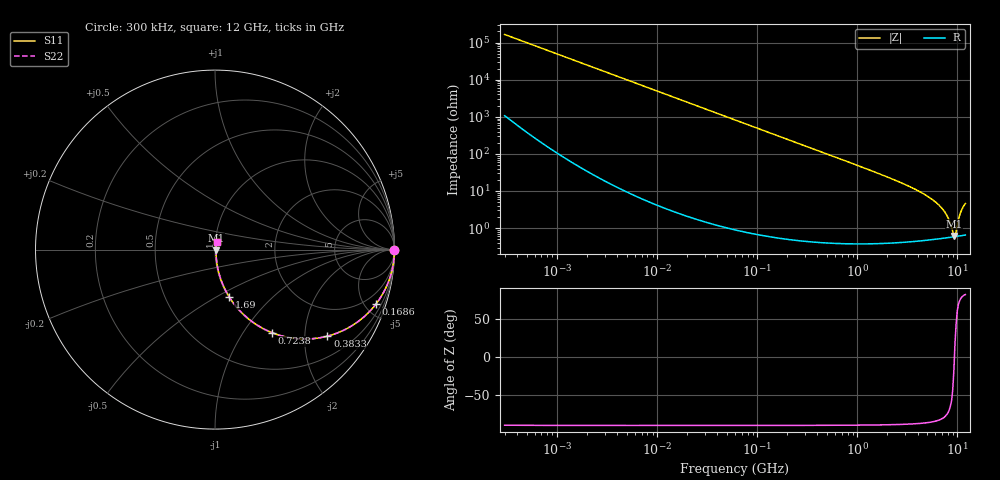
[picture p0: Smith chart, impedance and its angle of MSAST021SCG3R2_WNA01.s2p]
! MSAST021SCG3R2_WNA01  S-PARAMETER MODEL  ( General Type )
! Model Generated by TAIYO YUDEN Corporation (http://www.ty-top.com)
! Version 2.0
! TAIYO YUDEN Control No. 181101
! Copyright(c) 2015 TAIYO YUDEN CO.,LTD. All Rights Reserved.
! Product Description (link to TY-COMPAS)
! https://ds.yuden.co.jp/TYCOMPAS/or/detail?pn=MSAST021SCG3R2BWNA01&u=M
! Products Name : Multilayer Ceramic Capacitors
! Characteristics :
!  Capacitance : 3.2 pF , Rated Voltage : 25V , TCC : CG / C0G
!  Case Size : 0.25 x 0.125 / 0.0098 x 0.0049 [mm/inch] , Thickness : 0.125 / 0.0049 [mm/inch]
!  (Conditions: Temperature = 25 degC , DC Bias Current/Voltage = 0A / 0V)
! External Node Assignments :
!  1  o---| |---o  2
! GND o---------o GND
! Frequency Range : 0.3MHz  -  12000MHz  [ 401 STEP ]
# MHz S RI R 50
! Freq[MHz].  S11 Real  S11 Imag  S21 Real  S21 Imag  S12 Real  S12 Imag  S22 Real  S22 Imag
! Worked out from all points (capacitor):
!   401 points, 300 kHz to 12 GHz, reference 50 ohm
!   read as one part in series: C = 3.2 pF near 316.3 kHz
!   lowest |Z| = 613 mohm at 9.207 GHz (marker M1)
!   series resonance near 9.326 GHz, so ESL is about 91 pH
!   S11 on the Smith chart (normalised r, x): 300 kHz: open; 168.6 MHz: 1.01, -5.90; 383.3 MHz: 1.01, -2.59; 723.8 MHz: 1.01, -1.37; 1.69 GHz: 1.01, -0.57; 12 GHz: 1.01, +0.09
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0.3  1 -0.000603  4.27e-06 0.000603  4.27e-06 0.000603  1 -0.000603
1.769972  1 -0.00356  1.79e-05 0.00356  1.79e-05 0.00356  1 -0.00356
10.44266  0.9995 -0.021  0.000458 0.021  0.000458 0.021  0.9995 -0.021
60  0.9855 -0.1189  0.0145 0.1189  0.0145 0.1189  0.9855 -0.1189
168.5979  0.8964 -0.3038  0.1036 0.3038  0.1036 0.3038  0.8964 -0.3038
353.9943  0.6627 -0.4713  0.3373 0.4713  0.3373 0.4713  0.6627 -0.4713
383.2761  0.6263 -0.4822  0.3737 0.4822  0.3737 0.4822  0.6263 -0.4822
723.8279  0.3192 -0.4634  0.6808 0.4634  0.6808 0.4634  0.3192 -0.4634
1105.905  0.1667 -0.3685  0.8333 0.3685  0.8333 0.3685  0.1667 -0.3685
1689.663  0.0783 -0.262  0.9217 0.262  0.9217 0.262  0.0783 -0.262
2088.533  0.0524 -0.2143  0.9476 0.2143  0.9476 0.2143  0.0524 -0.2143
3944.255  0.0152 -0.1031  0.9848 0.1031  0.9848 0.1031  0.0152 -0.1031
6026.253  0.00749 -0.0499  0.9925 0.0499  0.9925 0.0499  0.00749 -0.0499
6879.757  0.00647 -0.0353  0.9935 0.0353  0.9935 0.0353  0.00647 -0.0353
7648.807  0.00598 -0.0236  0.994 0.0236  0.994 0.0236  0.00598 -0.0236
8281.503  0.0058 -0.0149  0.9942 0.0149  0.9942 0.0149  0.0058 -0.0149
8966.534  0.00578 -0.00541  0.9942 0.00541  0.9942 0.00541  0.00578 -0.00541
9207.246  0.00581 -0.00185  0.9942 0.00185  0.9942 0.00185  0.00581 -0.00185
9708.23  0.00597 0.00569  0.994 -0.00569  0.994 -0.00569  0.00597 0.00569
10511.28  0.00657 0.0208  0.9934 -0.0208  0.9934 -0.0208  0.00657 0.0208
11083.22  0.00724 0.031  0.9928 -0.031  0.9928 -0.031  0.00724 0.031
12000  0.00849 0.0446  0.9915 -0.0446  0.9915 -0.0446  0.00849 0.0446
